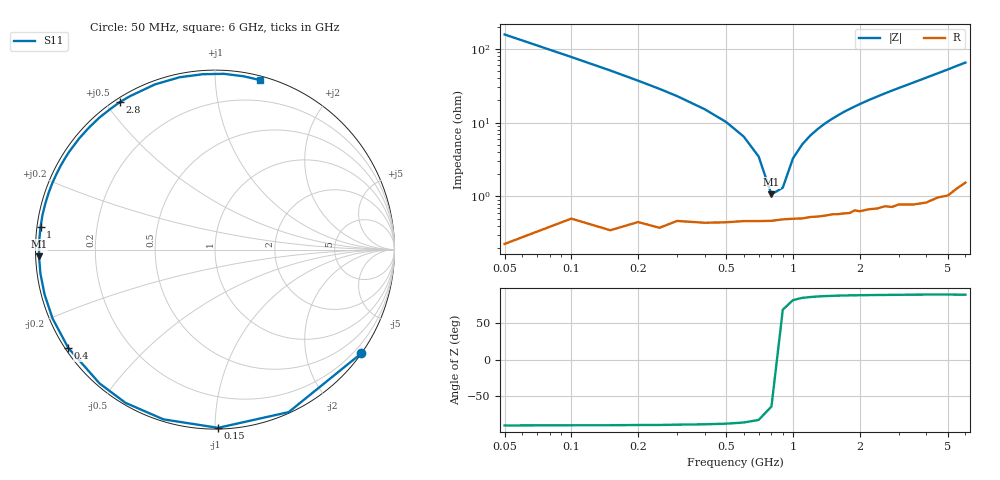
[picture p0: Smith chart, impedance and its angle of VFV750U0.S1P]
! Infineon Technologies  Discrete & RF Semiconductors
! BBY 58-03
! Si Tuning Diode in SOD323
! VR = 0.75 V
! S-Parameters:  June  1999
# GHz  S  MA  R  50
!  f  S11
! GHz  MAG  ANG
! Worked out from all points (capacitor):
!   34 points, 50 MHz to 6 GHz, reference 50 ohm
!   read as one part to ground: C = 20.2 pF near 50 MHz
!   lowest |Z| = 1.07 ohm at 800 MHz (marker M1)
!   series resonance near 844 MHz, so ESL is about 1.8 nH
!   S11 on the Smith chart (normalised r, x): 50 MHz: 0.00, -3.13; 150 MHz: 0.01, -1.02; 400 MHz: 0.01, -0.30; 1 GHz: 0.01, +0.06; 2.8 GHz: 0.01, +0.54; 6 GHz: 0.03, +1.30
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0.05  0.9992 -35.4
0.1  0.9941 -65.6
0.15  0.9932 -89.0
0.2  0.9885 -106.9
0.25  0.9887 -120.3
0.3  0.9847 -130.8
0.4  0.984 -146.2
0.5  0.983 -157.0
0.6  0.9819 -165.3
0.7  0.9817 -172.1
0.8  0.9815 -177.8
1  0.9803 172.6
1.1  0.9803 168.5
1.3  0.9794 161.2
1.4  0.979 157.8
1.6  0.9786 151.7
1.8  0.9785 146.0
2  0.9779 140.8
2.2  0.9772 135.9
2.4  0.9774 131.4
2.8  0.978 122.9
3  0.9772 119.0
3.5  0.9793 110.0
4  0.9803 101.6
4.5  0.9795 94.0
5  0.9806 87.1
5.5  0.9787 80.6
6  0.9774 75.0
